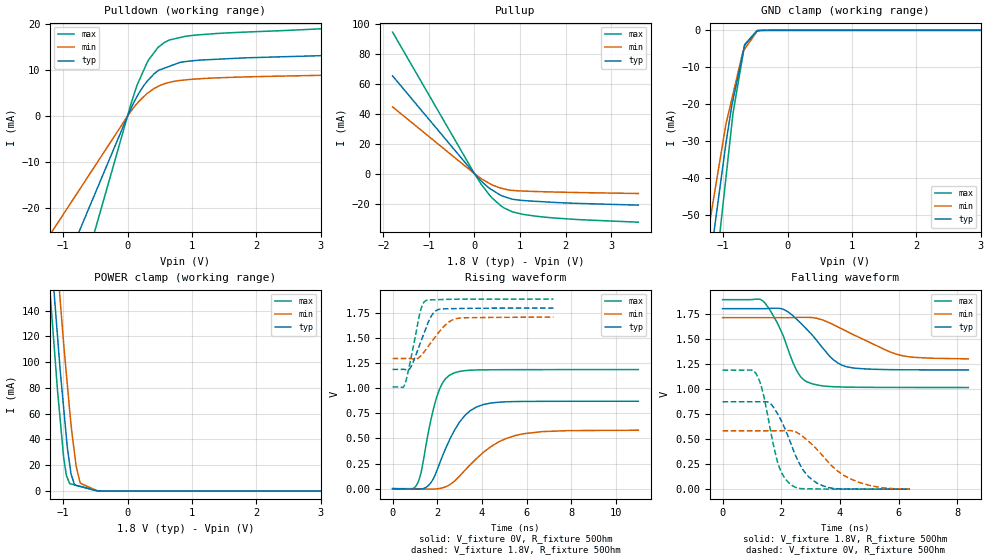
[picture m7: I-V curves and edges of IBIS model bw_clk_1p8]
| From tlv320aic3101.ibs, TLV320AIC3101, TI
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|   bw_clk_1p8 Model
[Model]   bw_clk_1p8
Model_type   I/O
Polarity   Non-Inverting
Enable   Active-Low
Vinl = 0.54
Vinh = 1.26
Vmeas = 0.9
Vref = 0.9
Cref = 2pF
Rref = 50
|   typ   min   max
|   (nom PVT)   (fast PVT)   (slow PVT)
 C_comp   1.361e-12   1.351e-12   1.385e-12
| Where nom  PVT is Nominal Process, 1.8V, 27C
|   Fast PVT is Strong Process,  1.89V, -40C
|   Slow PVT is Weak Process,   1.71V, 105C
[Voltage Range]   1.8   1.71   1.89
|Ambient Temperature   25   85   -40
|Junction Temperature
[Temperature Range]   27   105   -40
[Pullup Reference]   1.8   1.71   1.89
[Pulldown Reference]   0   0   0
[Power Clamp Reference]   1.8   1.71   1.89
[GND Clamp Reference]   0   0   0
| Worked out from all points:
|   slope of the pulldown table from 0 to 0.27 V, typ, clamps not added: 38.8 ohm
|   slope of the pullup table from 0 to 0.27 V, typ, clamps not added: 32.8 ohm
|   GND clamp passes 1 mA (typ) near -0.52 V on its own axis
|   falling waveform, V_fixture 1.8V, R_fixture 50Ohm: 20-80 % time 1.11ns typ, 1.74ns min, 759ps max; typ from 1.8 V to 1.19 V
|   rising waveform, V_fixture 0V, R_fixture 50Ohm: 20-80 % time 1.15ns typ, 1.79ns min, 690ps max; typ from 0 V to 0.871 V
|   rising waveform, V_fixture 1.8V, R_fixture 50Ohm: 20-80 % time 629ps typ, 873ps min, 469ps max; typ from 1.19 V to 1.8 V
|   falling waveform, V_fixture 0V, R_fixture 50Ohm: 20-80 % time 811ps typ, 1.29ns min, 525ps max; typ from 0.871 V to 0 V
[Pulldown]
|   Voltage   I(typ)   I(min)   I(max)
-1.8V     -59.89mA   -38.41mA   -88.18mA
-66.6mV   -2.216mA   -1.421mA   -3.263mA
51.03mV   1.569mA    1.01mA     2.575mA
145.5mV   4.212mA    2.715mA    6.623mA
252mV     6.622mA    4.23mA     9.986mA
302.4mV   7.55mA     4.897mA    11.57mA
470.6mV   9.821mA    6.44mA     14.86mA
574.6mV   10.42mA    7.046mA    16mA
655.8mV   10.84mA    7.342mA    16.54mA
817.2mV   11.67mA    7.747mA    17.05mA
1.139V    12.17mA    8.129mA    17.67mA
3.6V      13.41mA    9.027mA    19.33mA
[GND Clamp]
|   Voltage   I(typ)   I(min)   I(max)
-1.8V     -214.3mA   -124.8mA   -314.4mA
-1.416V   -95mA      -73.87mA   -121.3mA
-1.147V   -55.1mA    -45.4mA    -70.41mA
-1.138V   -53.96mA   -44.46mA   -68.74mA
-959.3mV  -30.91mA   -25.6mA    -40.31mA
-867.6mV  -20.57mA   -18.75mA   -25.7mA
-846.7mV  -18.82mA   -17.19mA   -22.43mA
-692.5mV  -6.208mA   -5.723mA   -6.628mA
-665.3mV  -4.021mA   -5.046mA   -3.834mA
-470.6mV  -78.13uA   -207.8uA   -26.68uA
-287.3mV  -491.1nA   -2.439uA   -14.54nA
3.6V      0A         0A         0A
[Pullup]
|   Voltage   I(typ)   I(min)   I(max)
-1.8V     65.23mA    44.56mA    94.44mA
0V        0A         0A         0A
151.2mV   -4.943mA   -3.327mA   -7.217mA
332.6mV   -9.769mA   -6.557mA   -14.34mA
574.6mV   -14.37mA   -9.577mA   -21.25mA
835.4mV   -16.98mA   -11.14mA   -25.46mA
1.058V    -17.83mA   -11.55mA   -27.07mA
1.382V    -18.48mA   -11.9mA    -28.45mA
2.268V    -19.79mA   -12.55mA   -30.57mA
3.6V      -20.92mA   -13.2mA    -32.33mA
[POWER Clamp]
|   Voltage   I(typ)   I(min)   I(max)
-1.8V     606.6mA    650.5mA    579.4mA
-1.217V   202.4mA    257.1mA    163mA
-1.159V   165.8mA    218.4mA    125.2mA
-1.089V   120.7mA    174.4mA    78.64mA
-1.048V   94.53mA    148.9mA    56.18mA
-990.4mV  63.47mA    113.3mA    25.31mA
-948.8mV  40.91mA    90.09mA    11.75mA
-897.8mV  20.26mA    61.68mA    5.644mA
-798.6mV  4.341mA    19.37mA    4.34mA
-735.3mV  3.513mA    5.976mA    3.508mA
-470.3mV  62.38uA    112uA      27.2uA
3.6V      0A         0A         0A
[Ramp]
R_load = 50
|   typ   min   max
dV/dt_r   0.522871/1.13704e-09   0.349397/1.78525e-09   0.712027/6.8694e-10
dV/dt_f   0.366668/1.11205e-09   0.247649/1.74541e-09   0.525797/7.57621e-10
[Falling Waveform]
V_fixture = 1.8V
V_fixture_min = 1.71V
V_fixture_max = 1.89V
R_fixture = 50Ohm
|   Time   V(typ)   V(min)   V(max)
0s        1.8V       1.71V      1.89V
1.394ns   1.8V       1.71V      1.872V
1.922ns   1.804V     1.71V      1.624V
2.552ns   1.688V     1.713V     1.17V
2.772ns   1.624V     1.714V     1.09V
3.046ns   1.54V      1.711V     1.052V
3.738ns   1.301V     1.646V     1.022V
4.218ns   1.221V     1.576V     1.018V
6.048ns   1.191V     1.337V     1.014V
8.378ns   1.189V     1.3V       1.014V
[Rising Waveform]
V_fixture = 0V
V_fixture_min = 0V
V_fixture_max = 0V
R_fixture = 50Ohm
|   Time   V(typ)   V(min)   V(max)
0s        1.077nV    21.47nV    568.4pV
1.106ns   -5.2mV     -679.9uV   47.72mV
1.292ns   -3.403mV   -2.913mV   177.1mV
1.932ns   150.6mV    -2.665mV   880.1mV
2.244ns   330.6mV    8.69mV     1.056V
2.588ns   503.7mV    43.53mV    1.136V
3.226ns   726.7mV    180.4mV    1.176V
3.75ns    813mV      298.5mV    1.183V
5.446ns   868mV      526.7mV    1.186V
11ns      871.5mV    582.3mV    1.187V
[Rising Waveform]
V_fixture = 1.8V
V_fixture_min = 1.71V
V_fixture_max = 1.89V
R_fixture = 50Ohm
|   Time   V(typ)   V(min)   V(max)
0s        1.189V     1.297V     1.014V
546ps     1.188V     1.297V     1.037V
814ps     1.211V     1.297V     1.291V
1.244ns   1.452V     1.319V     1.769V
1.372ns   1.528V     1.351V     1.847V
1.518ns   1.614V     1.395V     1.877V
1.728ns   1.718V     1.459V     1.883V
1.962ns   1.778V     1.528V     1.883V
2.804ns   1.795V     1.693V     1.888V
7.2ns     1.8V       1.71V      1.89V
[Falling Waveform]
V_fixture = 0V
V_fixture_min = 0V
V_fixture_max = 0V
R_fixture = 50Ohm
|   Time   V(typ)   V(min)   V(max)
0s        871.5mV    582.4mV    1.187V
1.144ns   871.3mV    582.4mV    1.151V
1.384ns   872.5mV    582.4mV    953.9mV
1.87ns    754.5mV    582.3mV    275.1mV
2.114ns   611.7mV    583.4mV    113.1mV
2.37ns    423.9mV    582.5mV    37.3mV
2.776ns   178.6mV    516mV      4.437mV
3.42ns    33.88mV    331.1mV    1.802mV
4.71ns    1.842mV    62.49mV    587.6uV
6.376ns   420.1uV    2.034mV    182.2uV
